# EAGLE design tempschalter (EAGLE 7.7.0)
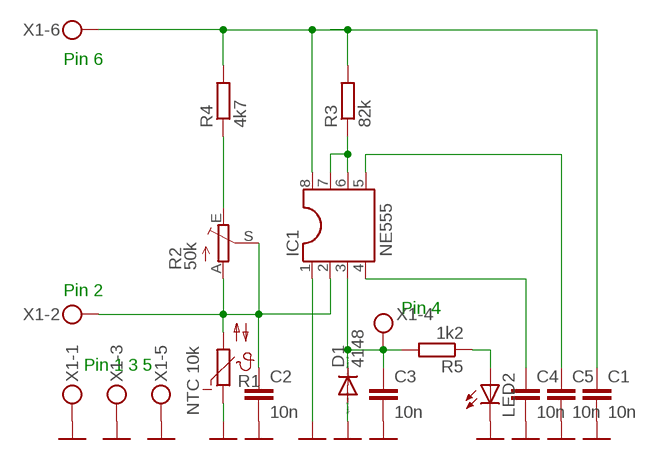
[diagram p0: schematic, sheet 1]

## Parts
C1  10n  C-EU050-024X044  [C050-024X044]
C2  10n  C-EU050-024X044  [C050-024X044]
C3  10n  C-EU050-024X044  [C050-024X044]
C4  10n  C-EU050-024X044  [C050-024X044]
C5  10n  C-EU050-024X044  [C050-024X044]
D1  4148  AA119  [DO07]
IC1  NE555  DIL8S  [SOCKET-08]
LED2  LED3MM  [LED3MM]
R1  NTC 10k  NTC642-6  [P642]
R2  50k  TRIM_EU-CA14H  [CA14H]
R3  82k  R-EU_0207/12  [0207/12]
R4  4k7  R-EU_0207/12  [0207/12]
R5  1k2  R-EU_0309/10  [0309/10]
X1  MKDSN1,5/6-5,08  [MKDSN1,5/6-5,08]

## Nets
0V: C1.2 C2.2 C3.2 C4.2 C5.2 D1.A IC1.1 LED2.K(C) R1.1 X1.1 X1.3 X1.5
N$1: C5.1 IC1.5
N$2: C4.1 IC1.4
N$3: IC1.6 IC1.7 R3.1
N$4: C1.1 IC1.8 R3.2 R4.2 X1.6
N$5: C2.1 IC1.2 R1.2 R2.A R2.S X1.2
N$6: R2.E R4.1
N$9: C3.1 D1.C IC1.3 R5.2 X1.4
N$12: LED2.A R5.1

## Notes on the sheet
- Pin 6
- Pin 2
- Pin 4
- Pin 1 3 5

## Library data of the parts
C1-C5 = resistor:C-EU: CAPACITOR, European symbol
D1 = diode:AA119: DIODE
IC1 = ic-package:DIL8: Dual In Line / Socket
LED2 = led:LED: LED
R1 = ptc-ntc:NTC642-6: PHILIPS NTC; OC_FARNELL: unknown; OC_NEWARK: unknown
R2 = pot:TRIM_EU-: POTENTIOMETER
R3 R4 = resistor:R-EU_: RESISTOR, European symbol
R5 = rcl:R-EU_: RESISTOR, European symbol
X1 = con-phoenix-508:MKDSN1,5/6-5,08: MKDSN 1,5/ 6-5,08 Printklemme Nennstrom: 13,5 A Nennspannung: 250 V Rastermaß: 5,08 mm Polzahl: 6 Anschlussart: Schraubanschluss Montage: Löten Anschlussrichtung Leiter/Platine: 0 ° Artikelnummer: 1729160 Source: http://eshop.phoenixcontact.com .. 1729160.pdf

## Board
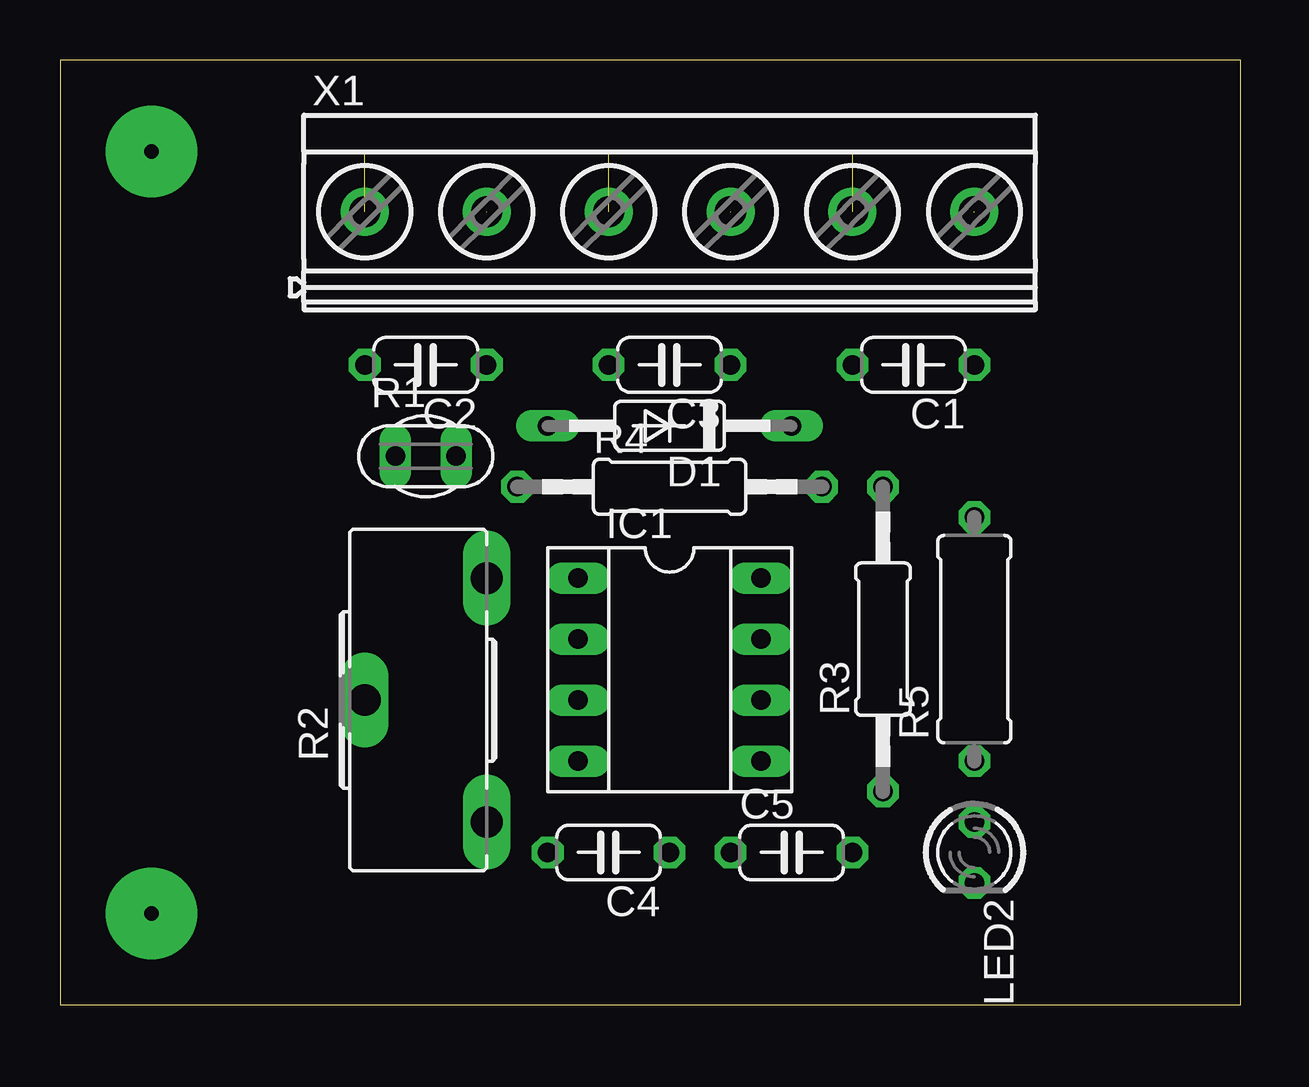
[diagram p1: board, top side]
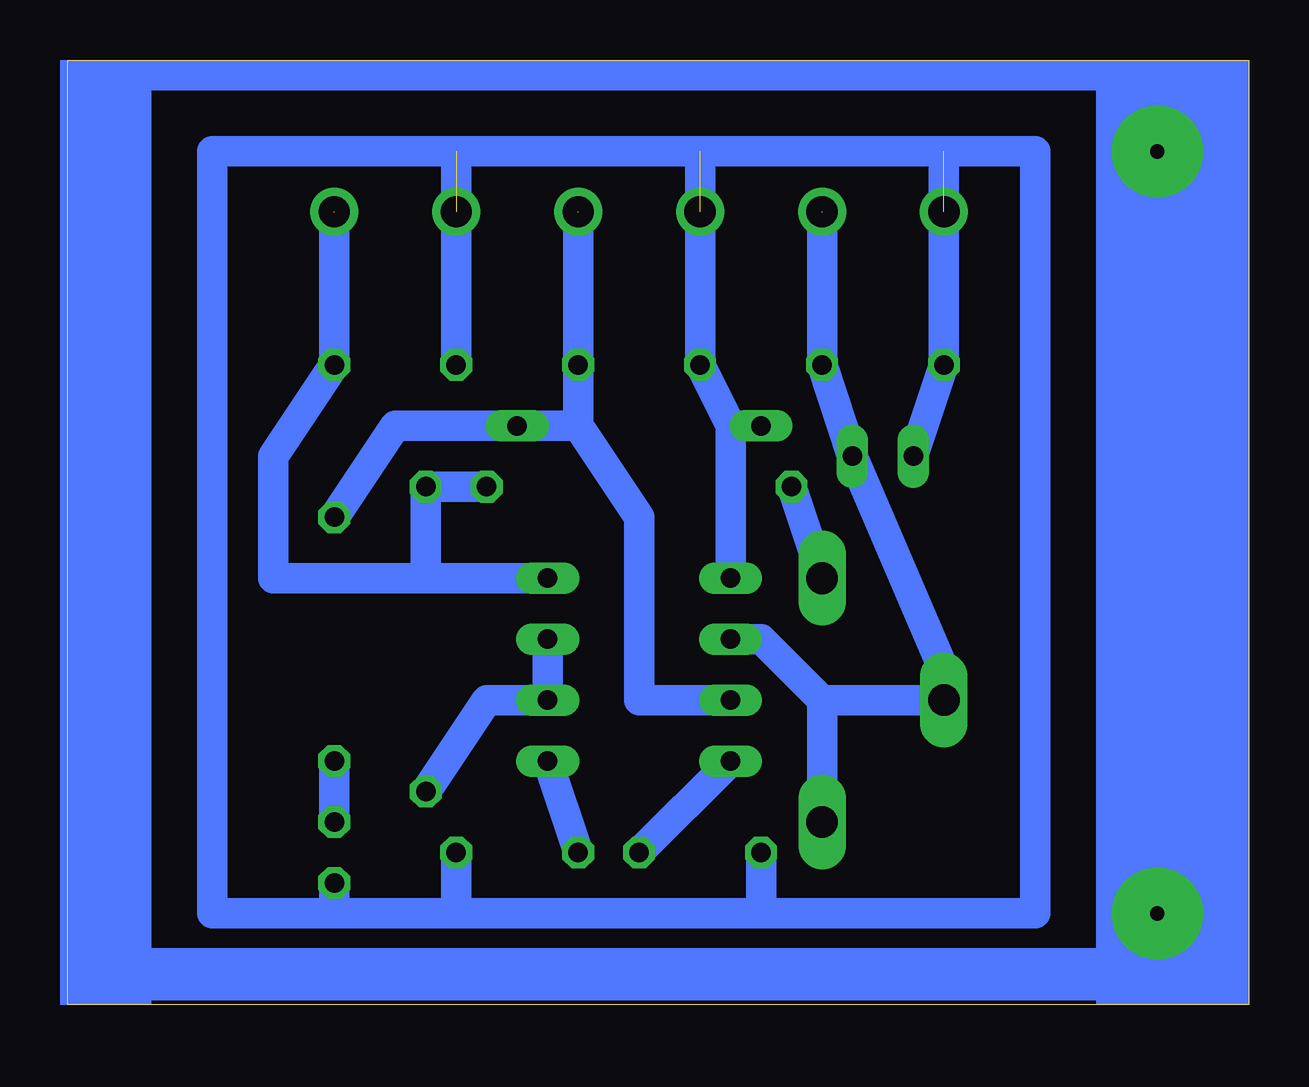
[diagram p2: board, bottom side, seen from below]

Size 49.2 x 39.36 mm. Coordinates in mm from the lower left corner, seen from the top.
Outline: 0,0 49.2,0 49.2,39.36 0,39.36 0,0
Copper layers (1*16): Top 0.035mm / dielectric 1.5mm / Bottom 0.035mm
Design rules "default": minimum track width 10mil, minimum drill 24mil, track to track 8mil, track to pad 8mil, pad to pad 8mil, via to via 8mil, smd to smd 8mil, copper to edge 40mil, drill to drill 8mil, minimum pad ring 10mil, minimum via ring 8mil, stop-mask expansion 4mil, vias tented up to drill 0mil, thermal gap 10mil

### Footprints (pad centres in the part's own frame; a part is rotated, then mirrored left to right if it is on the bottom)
C050-024X044 = drill 0.813 octagon: 1 -2.54,0; 2 2.54,0
DO35-10 = drill 0.813 long: A 5.08,0; C -5.08,0
SOCKET-08 = drill 0.813 long: 1 -3.81,-3.81; 2 -1.27,-3.81; 3 1.27,-3.81; 4 3.81,-3.81; 5 3.81,3.81; 6 1.27,3.81; 7 -1.27,3.81; 8 -3.81,3.81
LED3MM = drill 0.813 octagon: A -1.27,0; K 1.27,0
P642 = drill 0.813 long: 1 -1.27,0; 2 1.27,0
CA14H = drill 1.321 long: A -5.08,0; E 5.08,0; S 0,5.08
0207/12 = drill 0.813 octagon: 1 -6.35,0; 2 6.35,0
0309/10 = drill 0.813 octagon: 1 -5.08,0; 2 5.08,0
MKDSN1,5/6-5,08 = drill 1.3 pad 2: 1 -12.7,0.025; 2 -7.62,0.025; 3 -2.54,0.025; 4 2.54,0.025; 5 7.62,0.025; 6 12.7,0.025

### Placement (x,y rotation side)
C1  35.56,26.67 180 top
C2  15.24,26.67 180 top
C3  25.4,26.67 180 top
C4  22.86,6.35 180 top
C5  30.48,6.35 0 top
D1  4148  [DO35-10]  25.4,24.13 180 top
IC1  25.4,13.97 270 top
LED2  38.1,6.35 270 top
R1  15.24,22.86 0 top
R2  17.78,12.7 90 top
R3  34.29,15.24 90 top
R4  25.4,21.59 0 top
R5  38.1,15.24 90 top
X1  25.4,33.02 0 top

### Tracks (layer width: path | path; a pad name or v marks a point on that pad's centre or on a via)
0V  (3 unrouted)
  Bottom 1.27: 12.7,35.56 22.86,35.56 | 22.86,35.56 33.02,35.56 | 12.7,35.56 C2.2 R1.1 | 22.86,35.56 C3.2 21.59,24.13 | C1.2 33.02,35.56 | D1.A 21.59,24.13 | IC1.1 21.59,24.13 | 33.02,35.56 43.18,35.56 43.18,3.81 38.1,3.81 | 38.1,3.81 33.02,3.81 | 33.02,3.81 20.32,3.81 | 20.32,3.81 8.89,3.81 8.89,35.56 12.7,35.56 | C4.2 20.32,3.81 | C5.2 33.02,3.81 | LED2.K 38.1,3.81
N$1
  Bottom 1.27: C5.1 IC1.5
N$2
  Bottom 1.27: C4.1 IC1.4
N$3
  Bottom 1.27: R3.1 31.75,12.7 IC1.6 IC1.7
N$4  (1 unrouted)
  Bottom 1.27: 38.1,33.02 C1.1 40.64,22.86 40.64,17.78 34.29,17.78 | IC1.8 34.29,17.78 | 34.29,17.78 R3.2 R4.2
N$5  (1 unrouted)
  Bottom 1.27: 17.78,33.02 C2.1 R1.2 12.7,13.97 R2.S 17.78,12.7 | 17.78,12.7 20.32,15.24 IC1.2 | R2.A 17.78,12.7
N$6
  Bottom 1.27: R4.1 R2.E
N$7
  Bottom 2.184: 6.35,1.27 46.99,1.27
N$8  (via drill 0.6 pad 3.81)
  other vias: 3.81,3.81
N$9  (1 unrouted)
  Bottom 1.27: 27.94,33.02 C3.1 27.94,24.13 | 27.94,24.13 D1.C 35.56,24.13 R5.2 | IC1.3 25.4,12.7 25.4,20.32 27.94,24.13
N$10  (via drill 0.6 pad 3.81)
  other vias: 3.81,35.56
N$12
  Bottom 1.27: R5.1 LED2.A
(copper drawn outside any net)
  shapes: Bottom area x3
